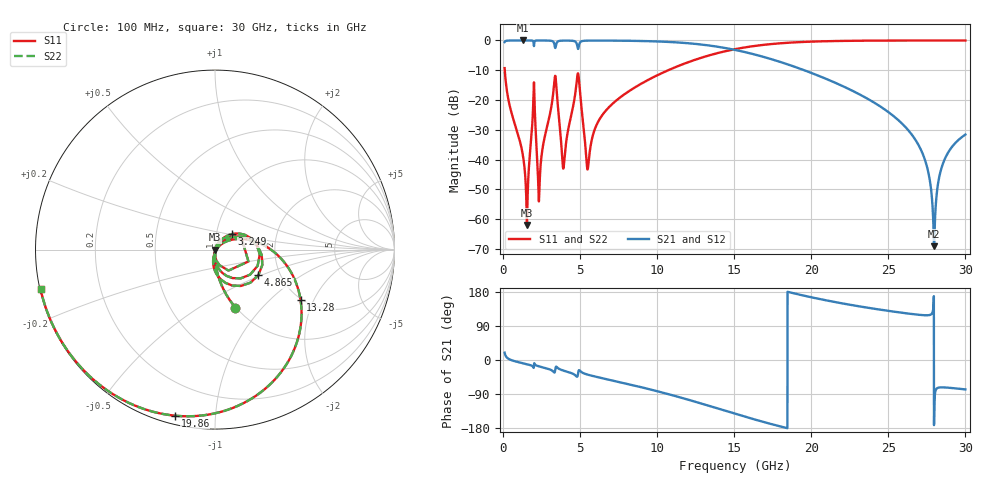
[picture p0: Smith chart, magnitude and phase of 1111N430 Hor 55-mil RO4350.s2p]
# GHz S MA R 50
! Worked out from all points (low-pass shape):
!   3201 points, 100 MHz to 30 GHz, reference 50 ohm
!   highest |S21| = -0.01 dB at 1.268 GHz (marker M1); lowest = -69.1 dB at 27.97 GHz (marker M2)
!   |S21| within 3 dB of the highest: start of sweep to 14.89 GHz
!   lowest |S11| = -61.9 dB at 1.548 GHz (marker M3), VSWR 1.00, Z = 50.1 - j0.0227 ohm
!   |S11| at or under -10 dB: 109.4 MHz to 10.72 GHz (10.61 GHz wide, 196 % of centre)
!   |S22| runs from -61.9 to 0.0 dB; largest |S21 - S12| = 0
!   S11 on the Smith chart (normalised r, x): 100 MHz: 0.99, -0.73; 3.249 GHz: 1.18, +0.21; 4.865 GHz: 1.55, -0.48; 13.28 GHz: 1.97, -1.59; 19.86 GHz: 0.04, -0.79; 30 GHz: 0.00, -0.11
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0.1  0.3429 -70.6  0.9392 19.3  0.9392 19.3  0.3429 -70.6
1.267969  0.01255 -95.7  0.9992 -8.4  0.9992 -8.4  0.01255 -95.7
1.548281  0.0008001 -16.5  0.999 -11.1  0.999 -11.1  0.0008001 -16.5
1.950063  0.0762 55.0  0.975 -18.2  0.975 -18.2  0.0762 55.0
2.370531  0.00404 46.2  0.9979 -17.2  0.9979 -17.2  0.00404 46.2
3.248844  0.1265 42.9  0.9553 -30.1  0.9553 -30.1  0.1265 42.9
3.454406  0.1725 -62.7  0.8703 -17.6  0.8703 -17.6  0.1725 -62.7
3.930938  0.007429 -2.2  0.9929 -28.1  0.9929 -28.1  0.007429 -2.2
4.865312  0.2805 -30.5  0.7198 -35.8  0.7198 -35.8  0.2805 -30.5
5.089563  0.07381 -98.1  0.9673 -32.0  0.9673 -32.0  0.07381 -98.1
5.510031  0.007258 -10.2  0.993 -38.9  0.993 -38.9  0.007258 -10.2
6.612594  0.06378 37.8  0.9944 -49.6  0.9944 -49.6  0.06378 37.8
10.06978  0.2646 6.3  0.9604 -83.1  0.9604 -83.1  0.2646 6.3
13.28403  0.5525 -30.4  0.8279 -120.0  0.8279 -120.0  0.5525 -30.4
15.05  0.7135 -52.1  0.694 -141.7  0.694 -141.7  0.7135 -52.1
19.86203  0.9519 -103.6  0.2941 166.8  0.2941 166.8  0.9519 -103.6
20.03956  0.9555 -105.2  0.2824 165.2  0.2824 165.2  0.9555 -105.2
25.01978  0.995 -141.0  0.06216 129.6  0.06216 129.6  0.995 -141.0
27.16884  0.9969 -153.1  0.01359 118.6  0.01359 118.6  0.9969 -153.1
27.97241  0.9969 -157.3  0.0003507 -148.2  0.0003507 -148.2  0.9969 -157.3
28.58909  0.9969 -160.4  0.009173 -72.3  0.009173 -72.3  0.9969 -160.4
30  0.9966 -167.2  0.02626 -77.6  0.02626 -77.6  0.9966 -167.2
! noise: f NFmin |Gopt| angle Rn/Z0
0.1  0.0006449  0.7278  1.791  0.0004712
3.417  0.1264  0.9471  24.37  0.5122
6.743  0.01896  0.4866  45.74  0.005479
10.06  0.02418  0.4448  62.12  0.0056
13.39  0.03504  0.5089  77.04  0.008097
16.7  0.05518  0.6295  93.6  0.01386
20.03  0.09982  0.7721  112.7  0.02846
23.35  0.2294  0.8939  132.3  0.07828
26.67  1.132  0.9772  150.7  0.7325
30  1.019  0.9739  167.1  0.1151
